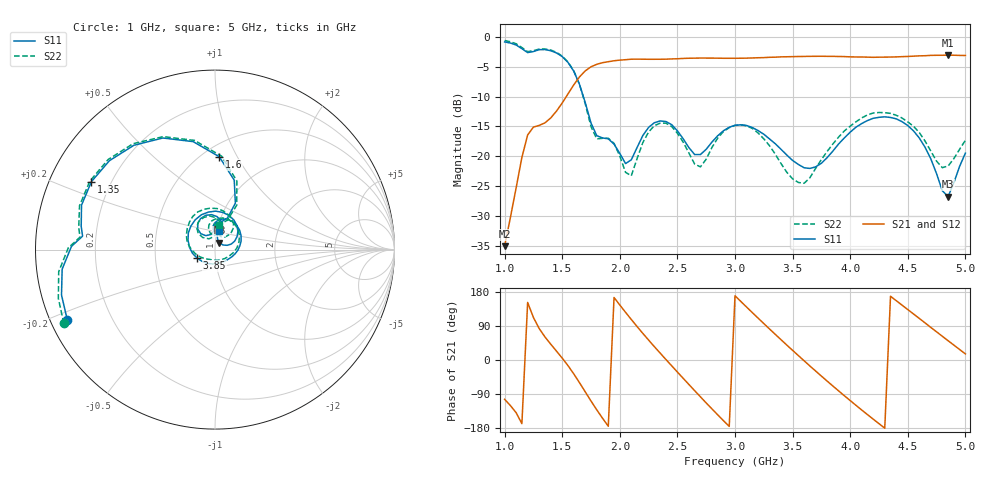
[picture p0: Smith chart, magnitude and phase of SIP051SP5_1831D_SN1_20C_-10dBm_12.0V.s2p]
# GHz  S  dB  R  50
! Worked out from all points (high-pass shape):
!   81 points, 1 GHz to 5 GHz, reference 50 ohm
!   highest |S21| = -3.04 dB at 4.85 GHz (marker M1); lowest = -35.1 dB at 1 GHz (marker M2)
!   |S21| within 3 dB of the highest: 1.682 GHz to end of sweep
!   lowest |S11| = -26.8 dB at 4.85 GHz (marker M3), VSWR 1.10, Z = 52.4 + j4.06 ohm
!   |S11| at or under -10 dB: 1.684 GHz to end of sweep
!   |S22| runs from -24.5 to -0.6 dB; largest |S21 - S12| = 0.0027
!   S11 on the Smith chart (normalised r, x): 1 GHz: 0.05, -0.22; 1.35 GHz: 0.13, +0.25; 1.6 GHz: 0.60, +0.85; 3.85 GHz: 0.81, -0.08; 5 GHz: 1.02, +0.21
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1  -0.81 -154.7  -35.09 -103.7  -35.05 -103.7  -0.56 -154.0
1.2  -2.60 174.2  -16.42 151.8  -16.43 151.9  -2.44 174.8
1.35  -2.09 151.2  -14.39 61.0  -14.39 60.8  -1.99 151.3
1.6  -5.71 87.4  -8.03 -36.4  -8.01 -36.4  -5.65 85.9
1.7  -10.98 66.3  -5.67 -84.0  -5.67 -84.1  -11.19 63.9
1.85  -16.92 90.0  -4.30 -153.6  -4.29 -153.7  -16.98 91.9
1.95  -17.96 90.6  -3.97 164.9  -3.98 165.0  -17.82 87.3
2.15  -18.53 131.8  -3.70 88.3  -3.69 88.3  -20.39 135.4
2.35  -14.07 105.1  -3.72 18.3  -3.71 18.2  -14.44 109.6
2.5  -15.73 78.8  -3.63 -31.8  -3.62 -31.8  -16.14 79.4
2.65  -19.71 80.1  -3.53 -81.0  -3.53 -81.0  -21.32 78.6
2.85  -16.55 90.5  -3.54 -144.7  -3.55 -144.7  -16.95 103.6
3  -14.79 67.1  -3.55 169.6  -3.55 169.6  -14.84 76.3
3.3  -17.10 8.5  -3.39 81.8  -3.39 81.8  -18.23 4.3
3.5  -20.70 -34.4  -3.28 25.4  -3.28 25.4  -23.79 -62.3
3.7  -21.77 -100.3  -3.22 -29.1  -3.22 -29.0  -22.04 -142.3
3.85  -19.12 -155.1  -3.23 -68.7  -3.24 -68.8  -17.93 -177.8
4.05  -15.12 147.8  -3.34 -119.5  -3.33 -119.5  -14.22 142.6
4.35  -13.49 78.4  -3.35 168.2  -3.36 168.2  -12.80 87.1
4.6  -16.94 30.3  -3.15 109.6  -3.15 109.5  -16.02 49.7
4.85  -26.76 57.4  -3.04 50.8  -3.04 50.9  -21.63 73.5
5  -19.48 78.5  -3.09 16.1  -3.10 16.2  -17.31 80.9
